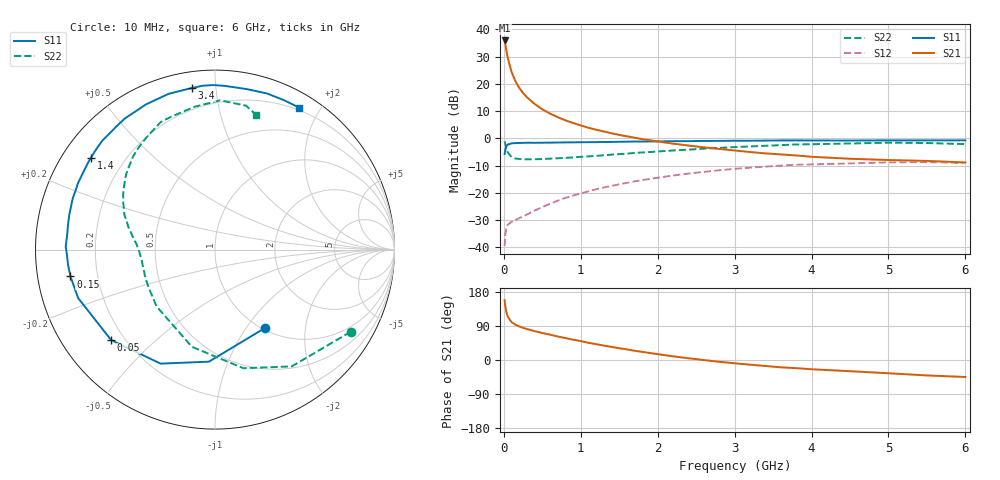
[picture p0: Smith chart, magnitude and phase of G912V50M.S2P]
! SIEMENS Small Signal Semiconductors
! BFG235
! Si NPN RF Bipolar Junction Transistor in SOT223
! VCE = 12 V  IC = 50 mA
! Common Emitter S-Parameters:  July  1994
# GHz  S  MA  R  50
!  f  S11  S21  S12  S22
! GHz  MAG  ANG  MAG  ANG  MAG  ANG  MAG  ANG
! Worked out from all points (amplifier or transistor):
!   40 points, 10 MHz to 6 GHz, reference 50 ohm
!   highest |S21| = 35.9 dB at 10 MHz (marker M1)
!   |S21| within 3 dB of that: start of sweep to 29.14 MHz
!   unconditionally stable (mu >= 1): 514.4 MHz to 1.317 GHz
!   at 200 MHz: K = 0.65, MSG = 23.9 dB, |S12| = -29.3 dB
!   at 1.5 GHz: K = 0.97, MSG = 9.1 dB, |S12| = -16.9 dB
!   at 6 GHz: K = 0.92, MSG = 0.1 dB, |S12| = -9.0 dB
!   S11 on the Smith chart (normalised r, x): 10 MHz: 1.03, -1.23; 50 MHz: 0.15, -0.37; 150 MHz: 0.10, -0.09; 1.4 GHz: 0.08, +0.33; 3.4 GHz: 0.08, +0.86; 6 GHz: 0.17, +1.74
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0.01  0.5179 -57.3  62.57 157.8  0.0105 68.5  0.8837 -31.2
0.02  0.6253 -93.1  52.53 140.9  0.0175 53.8  0.7786 -56.7
0.03  0.7039 -115.5  43.59 128.9  0.0219 45.6  0.6798 -76.5
0.05  0.7673 -138.9  30.49 114.7  0.0259 34.3  0.5565 -103.4
0.1  0.8089 -160.5  16.61 100.1  0.0293 30.3  0.4541 -135.8
0.15  0.8191 -169.5  11.23 93.1  0.0314 33.4  0.426 -150.3
0.2  0.8232 -174.1  8.435 88.5  0.0344 36.7  0.4183 -158.4
0.25  0.8255 -178.2  6.797 84.8  0.0368 40.2  0.4131 -163.5
0.3  0.8321 178.9  5.68 81.8  0.04 43.5  0.4125 -167.4
0.4  0.8277 173.6  4.273 76.1  0.0474 48.5  0.4128 -172.5
0.5  0.8312 169.9  3.408 71.2  0.0547 51.5  0.4179 -176.0
0.6  0.8347 166.4  2.845 66.9  0.0629 53.8  0.4235 -179.0
0.7  0.8381 162.8  2.448 62.1  0.0718 55.3  0.4312 178.5
0.9  0.8435 157.1  1.913 53.7  0.0889 55.5  0.4468 174.4
1.1  0.85 150.7  1.563 45.3  0.1067 54.8  0.4676 170.4
1.4  0.8597 143.4  1.24 34.5  0.1339 52.1  0.502 164.8
2.2  0.8867 124.4  0.8 9.7  0.2077 39.6  0.5993 148.6
3.2  0.9053 102.4  0.561 -12.3  0.2897 19.8  0.7104 126.8
3.4  0.9094 98.2  0.53 -15.8  0.3027 15.5  0.7302 121.9
4.5  0.9116 78.5  0.422 -29.6  0.3467 -6.7  0.8039 98.1
5.5  0.9168 65.2  0.385 -40.7  0.3654 -25.7  0.8203 77.8
6  0.9195 59.4  0.361 -44.8  0.3538 -32.5  0.7838 72.9
